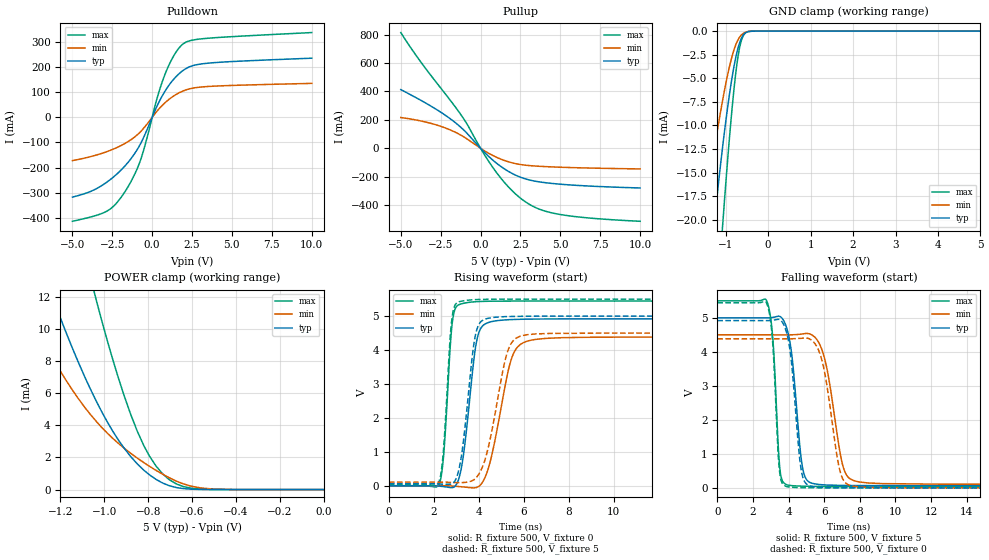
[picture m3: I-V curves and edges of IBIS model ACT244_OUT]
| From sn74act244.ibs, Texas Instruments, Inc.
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[Model]   ACT244_OUT
Model_type  3-state
Enable   Active-Low
Vref =   0
Rref =   500
Cref =   50p
Vmeas =   1.5
| variable   typ   min   max
C_comp   6.21pF   5.55pF   7.05pF
| C_pullup   13.15pF   6.14pF   19.35pF
| C_pulldown   11.20pF   6.48pF   16.64pF
| C_tri-state   6.21pF   5.55pF   7.05pF
[Temperature Range]   40   100   -40
| Ambient temperature   25   85   -40
[Voltage range]   5   4.5   5.5
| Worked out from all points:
|   slope of the pulldown table from 0 to 0.75 V, typ, clamps not added: 7.64 ohm
|   slope of the pullup table from 0 to 0.75 V, typ, clamps not added: 9.15 ohm
|   GND clamp passes 1 mA (typ) near -0.65 V on its own axis
|   POWER clamp passes 1 mA (typ) near -0.80 V on its own axis
|   rising waveform, R_fixture 500, V_fixture 0: 20-80 % time 489ps typ, 782ps min, 298ps max; typ from 0 V to 4.92 V
|   falling waveform, R_fixture 500, V_fixture 5: 20-80 % time 512ps typ, 801ps min, 317ps max; typ from 5 V to 0.063 V
|   rising waveform, R_fixture 500, V_fixture 5: 20-80 % time 482ps typ, 774ps min, 292ps max; typ from 0.063 V to 5 V
|   falling waveform, R_fixture 500, V_fixture 0: 20-80 % time 490ps typ, 756ps min, 308ps max; typ from 4.92 V to 0 V
[GND Clamp]
| ACT244_OUT
|   Voltage   I(typ)   I(min)   I(max)
-5V       -263.4mA   -172.3mA   -333.6mA
-1.555V   -33.8mA    -21.36mA   -53.39mA
-1.505V   -31.3mA    -19.74mA   -49.78mA
-1.3V     -21.65mA   -13.45mA   -35.4mA
-1.25V    -19.45mA   -12.02mA   -32.02mA
-1.075V   -12.35mA   -7.382mA   -20.73mA
-1.055V   -11.6mA    -6.895mA   -19.51mA
-895mV    -6.193mA   -3.446mA   -10.42mA
-765mV    -2.832mA   -1.468mA   -4.517mA
-665mV    -1.141mA   -592.1uA   -1.585mA
-545mV    -219.7uA   -140.7uA   -227.2uA
5V        100.3nA    31.18uA    910.4nA
[POWER Clamp]
| ACT244_OUT
|   Voltage   I(typ)   I(min)   I(max)
-5V       301.4mA    205.9mA    466.9mA
-1.39V    18.12mA    12.2mA     34.24mA
-1.235V   11.94mA    8.167mA    23.48mA
-1.065V   6.3mA      4.701mA    13.3mA
-1.035V   5.458mA    4.217mA    11.7mA
-935mV    3.07mA     2.867mA    6.912mA
-850mV    1.604mA    1.964mA    3.643mA
-795mV    928.3uA    1.458mA    2.104mA
-705mV    248.2uA    744.4uA    629.4uA
-640mV    63.92uA    357.2uA    190.6uA
-505mV    1.994uA    34.9uA     10.07uA
-84.45fV  100.3nA    5.889nA    1.383uA
[Pulldown]
| ACT244_OUT
|   Voltage   I(typ)   I(min)   I(max)
-5V       -317mA     -172mA     -413.2mA
-3.785V   -292.5mA   -154.9mA   -394.9mA
-2.8V     -255.7mA   -135.4mA   -371.4mA
-2.245V   -227.2mA   -121.1mA   -341.5mA
-1.62V    -187mA     -100.6mA   -287.2mA
-700mV    -101.4mA   -55.19mA   -164.3mA
310mV     45.39mA    24.99mA    76.41mA
790mV     102.4mA    56.98mA    168.6mA
1.36V     152.3mA    85.38mA    245.4mA
1.925V    185.6mA    104.4mA    291.1mA
3.48V     215.1mA    122.5mA    314.3mA
10V       235mA      134.9mA    336.9mA
[Pullup]
| ACT244_OUT
|   Voltage   I(typ)   I(min)   I(max)
-5V       413.3mA    216.4mA    815.3mA
-3.725V   336.5mA    191.8mA    604.9mA
-1.745V   194.7mA    121.3mA    315.4mA
-930mV    114.7mA    71.39mA    185.1mA
125mV     -14.93mA   -9.324mA   -23.64mA
890mV     -95.25mA   -57.86mA   -154.5mA
1.705V    -160.4mA   -94.05mA   -267.5mA
2.52V     -205mA     -115.2mA   -353.4mA
3.525V    -234.2mA   -126.1mA   -422.1mA
4.76V     -251.2mA   -132.9mA   -462.2mA
6.775V    -266.3mA   -139.4mA   -491.5mA
10V       -280.2mA   -145.9mA   -515mA
[Ramp]
| ACT244_OUT
| variable   typ   min   max
dV/dt_r   2.98/4.97E-10   2.67/7.96E-10   3.29/3.10E-10
dV/dt_f   2.99/5.25E-10   2.66/8.15E-10   3.30/3.27E-10
R_load = 500
[Rising Waveform]
| ACT244_OUT
R_fixture =   500
C_fixture =   0
L_fixture =   0
V_fixture =   0
V_fixture_min = 0
V_fixture_max = 0
|   Time   V(typ)   V(min)   V(max)
0s        1.229nV    2.108nV    753.1pV
2.235ns   -11.03mV   407.8uV    48.28mV
2.44ns    -27.35mV   759.3uV    933.1mV
2.845ns   -52.25mV   -10.86mV   4.925V
3.46ns    1.699V     -45.71mV   5.395V
3.83ns    3.977V     -60.41mV   5.422V
4.095ns   4.649V     40.99mV    5.431V
5.485ns   4.899V     3.806V     5.442V
6.515ns   4.913V     4.312V     5.443V
50ns      4.918V     4.383V     5.443V
[Falling Waveform]
| ACT244_OUT
R_fixture =   500
C_fixture =   0
L_fixture =   0
V_fixture =   5
V_fixture_min = 4.5
V_fixture_max = 5.5
|   Time   V(typ)   V(min)   V(max)
0s        5V         4.5V       5.5V
2.805ns   4.999V     4.5V       5.463V
3.12ns    5.012V     4.5V       4.386V
3.525ns   5.038V     4.5V       519.4mV
3.97ns    4.568V     4.5V       81.41mV
4.78ns    616.3mV    4.526V     49.68mV
5.48ns    116.9mV    4.431V     44.25mV
7.08ns    72.12mV    595.1mV    41.31mV
7.955ns   67.88mV    174.4mV    40.98mV
50ns      63.36mV    104.1mV    40.77mV
[Rising Waveform]
| ACT244_OUT
R_fixture =   500
C_fixture =   0
L_fixture =   0
V_fixture =   5
V_fixture_min = 4.5
V_fixture_max = 5.5
|   Time   V(typ)   V(min)   V(max)
0s        63.36mV    104.1mV    40.77mV
2.215ns   55.07mV    104.4mV    93.71mV
2.42ns    45.14mV    104.8mV    980.3mV
2.82ns    65.94mV    96.34mV    4.999V
3.345ns   1.484V     96.17mV    5.454V
3.74ns    3.984V     159.2mV    5.481V
3.995ns   4.745V     337.4mV    5.489V
5.285ns   4.986V     3.97V      5.499V
6.15ns    4.995V     4.451V     5.5V
50ns      5V         4.5V       5.5V
[Falling Waveform]
| ACT244_OUT
R_fixture =   500
C_fixture =   0
L_fixture =   0
V_fixture =   0
V_fixture_min = 0
V_fixture_max = 0
|   Time   V(typ)   V(min)   V(max)
0s        4.918V     4.383V     5.443V
2.795ns   4.918V     4.383V     5.403V
3.105ns   4.928V     4.383V     4.32V
3.495ns   4.949V     4.382V     494.4mV
3.95ns    4.444V     4.383V     31.48mV
4.7ns     568.5mV    4.398V     6.189mV
5.29ns    42.24mV    4.346V     2.497mV
6.91ns    3.19mV     456.1mV    327uV
7.62ns    1.71mV     48.81mV    145.9uV
50ns      -6.149nV   -1.826nV   -3.133nV
